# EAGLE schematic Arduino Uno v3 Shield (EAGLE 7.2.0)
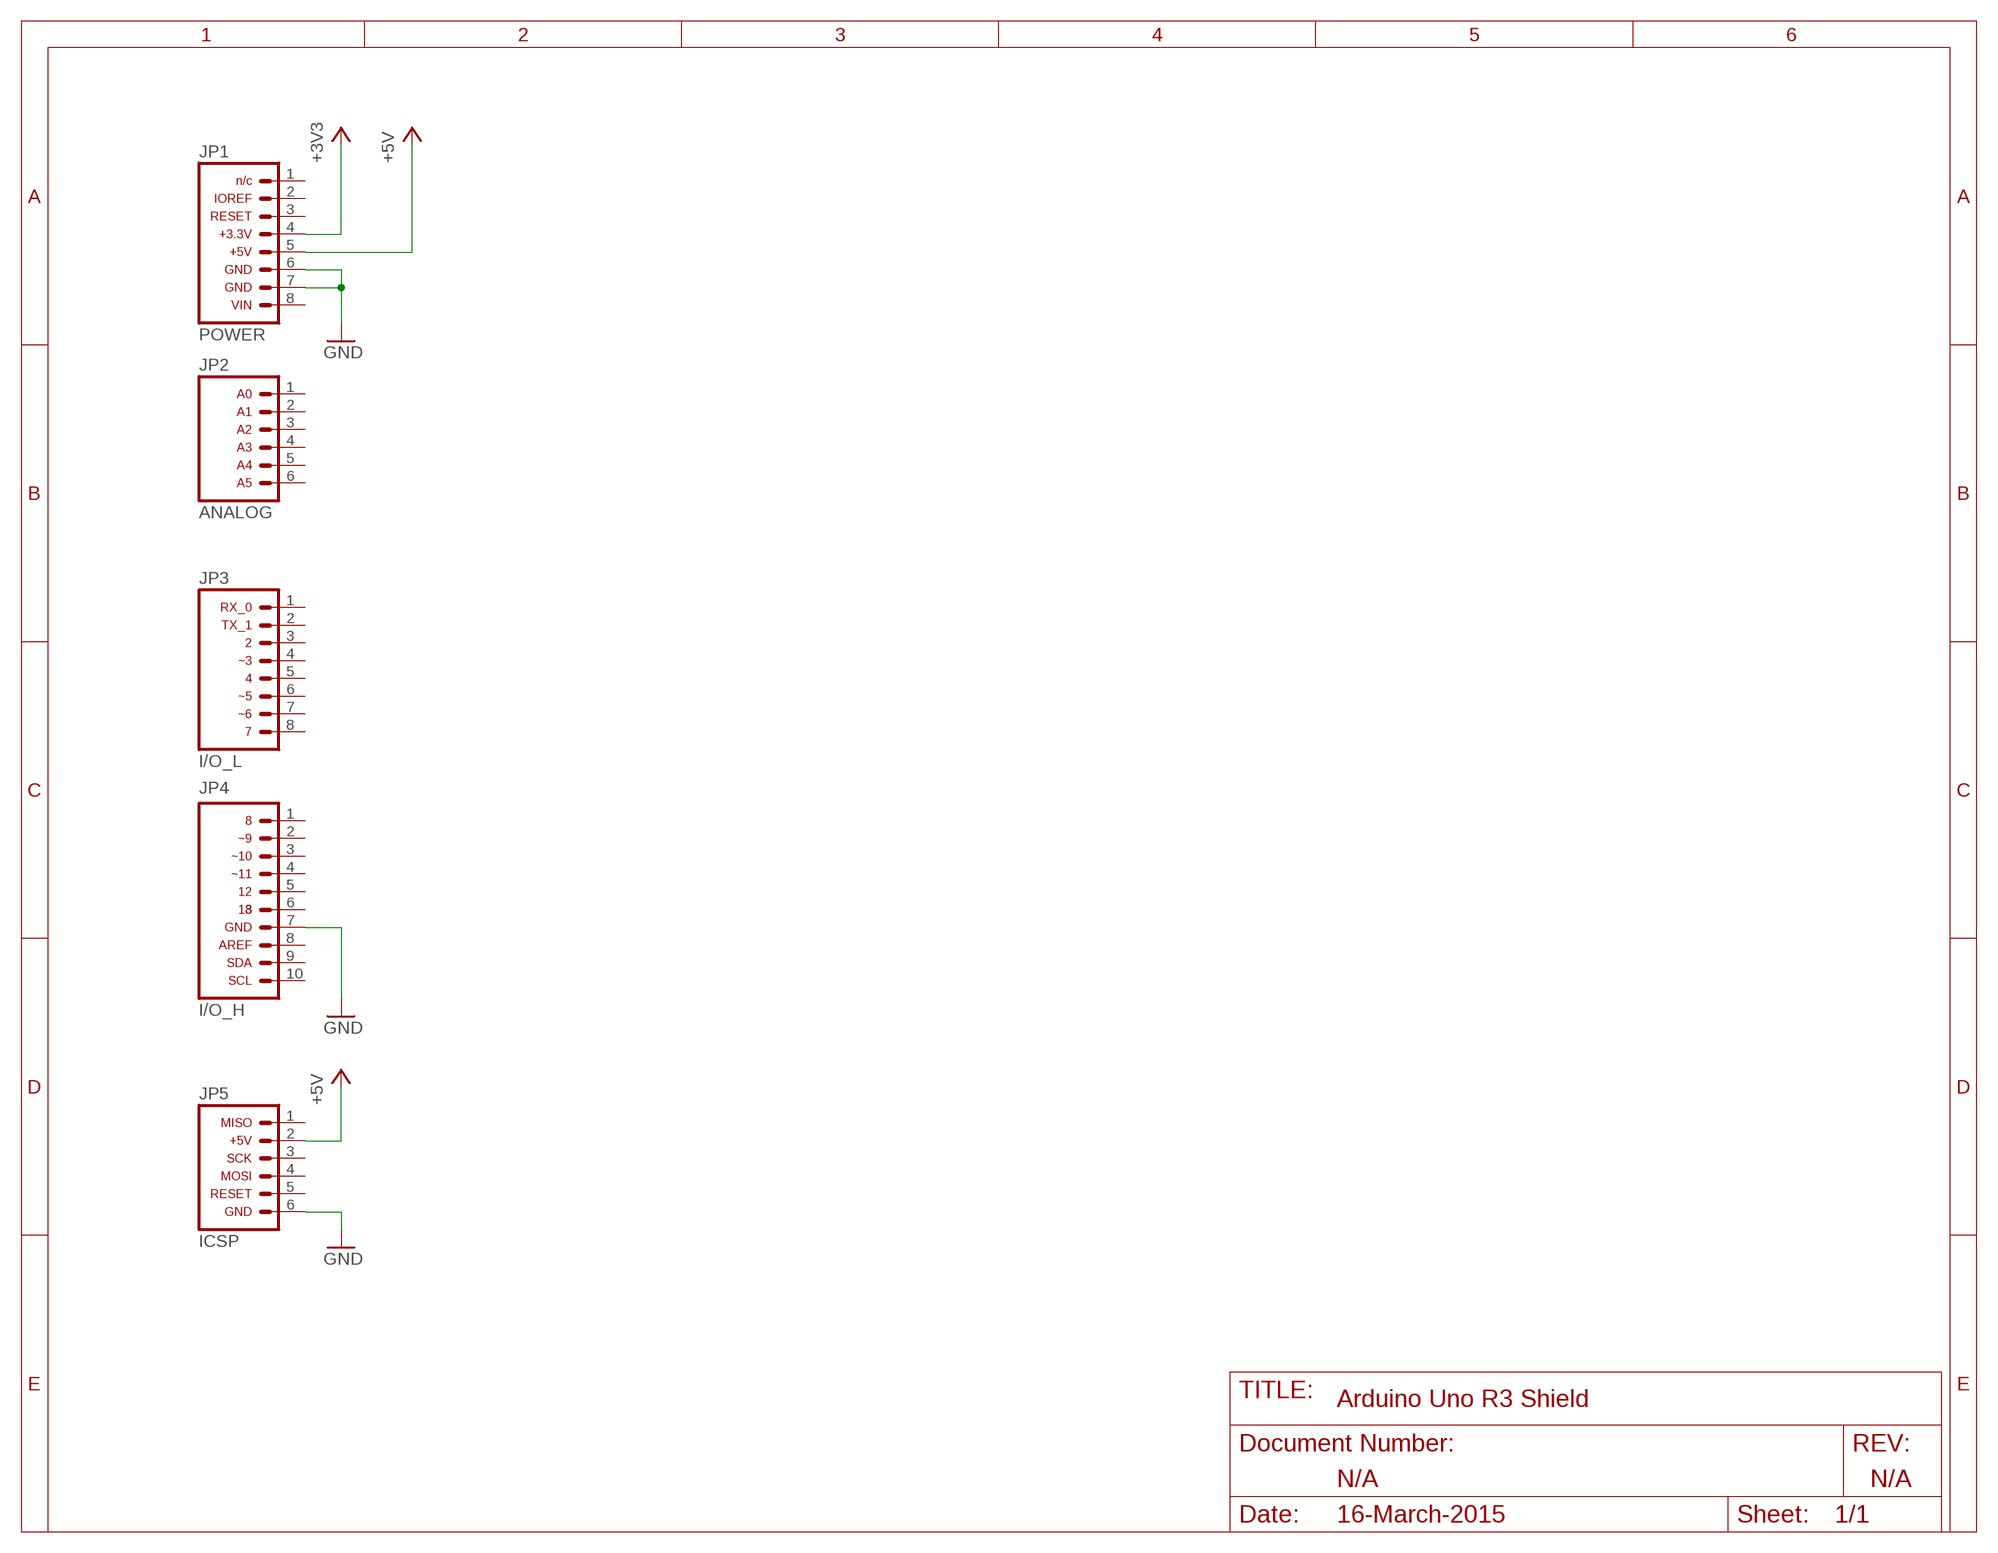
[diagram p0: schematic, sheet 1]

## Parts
JP1  ARDUINO_CONN-POWERSIP  [CONN-1X08]
JP2  ARDUINO_CONN-ANALOGSIP  [CONN-1X06]
JP3  ARDUINO_CONN-IO_LSIP  [CONN-1X08]
JP4  ARDUINO_CONN-IO_HSIP  [CONN-1X10]
JP5  ARDUINO_CONN-ICSP  [CONN-2X03]

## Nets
+3V3: JP1.4
+5V: JP1.5 JP5.2
GND: JP1.6 JP1.7 JP4.7 JP5.6
Unconnected: JP1.1 JP1.2 JP1.3 JP1.8 JP2.1 JP2.2 JP2.3 JP2.4 JP2.5 JP2.6 JP3.1 JP3.2 JP3.3 JP3.4 JP3.5 JP3.6 JP3.7 JP3.8 JP4.1 JP4.2 JP4.3 JP4.4 JP4.5 JP4.6 JP4.8 JP4.9 JP4.10 JP5.1 JP5.3 JP5.4 JP5.5

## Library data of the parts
JP1 = _Jim:ARDUINO_CONN-POWER: Arduino Power Header
JP2 = _Jim:ARDUINO_CONN-ANALOG: Arduino Analog I/O Header
JP3 = _Jim:ARDUINO_CONN-IO_L: Arduino Digital I/O [Low Byte] Header
JP4 = _Jim:ARDUINO_CONN-IO_H: Arduino Digital I/O [High Byte] Header
JP5 = _Jim:ARDUINO_CONN-ICSP: Header 6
